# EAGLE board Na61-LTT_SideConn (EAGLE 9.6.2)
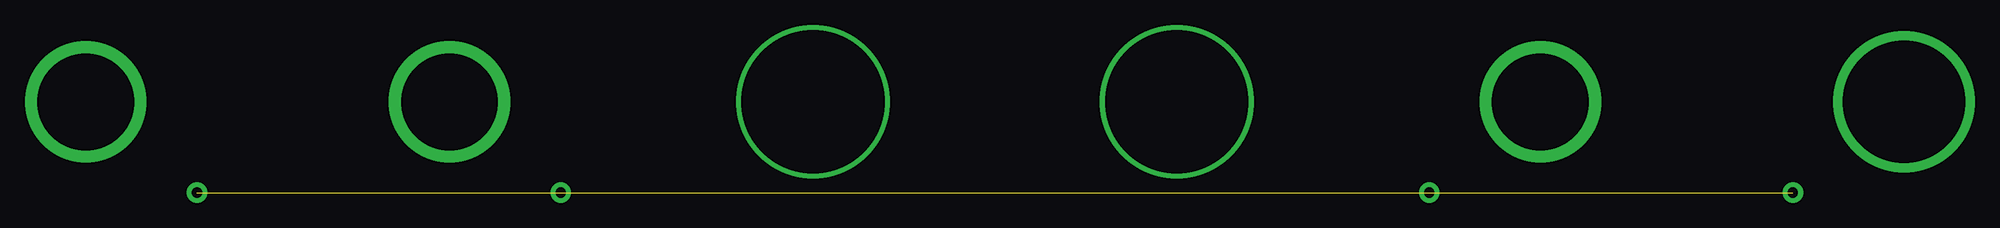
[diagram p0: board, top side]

No outline drawn. Coordinates in mm, seen from the top.
Copper layers (1*16): Top 0.035mm / dielectric 1.5mm / Bottom 0.035mm
Design rules "default": minimum track width 6mil, minimum drill 0.35mm, track to track 6mil, track to pad 6mil, pad to pad 6mil, via to via 6mil, smd to smd 6mil, copper to edge 40mil, drill to drill 6mil, minimum pad ring 10mil, minimum via ring 8mil, stop-mask expansion 4mil, vias tented up to drill 0mil, thermal gap 10mil

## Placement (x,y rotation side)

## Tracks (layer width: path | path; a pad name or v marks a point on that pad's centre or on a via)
S$1  (via drill 9.6 pad 12)
  other vias: -9,0
S$2  (via drill 1 pad 2)  (2 unrouted)
  other vias: 2,-9 160,-9 124,-9
S$3  (via drill 9.6 pad 12)
  other vias: 27,0
S$4  (via drill 14.2 pad 12)
  other vias: 63,0
S$5  (via drill 14.2 pad 12)
  other vias: 99,0
S$6  (via drill 9.6 pad 12)
  other vias: 135,0
S$7  (via drill 12.1 pad 14)
  other vias: 171,0
S$8  (via drill 1 pad 2)
  other vias: 38,-9

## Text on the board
tDocu: SenseW / SHV | FieldW / SHV | Gas / d14 | Gas / d14 | Cathode / SHV | GatingG / Lemo2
